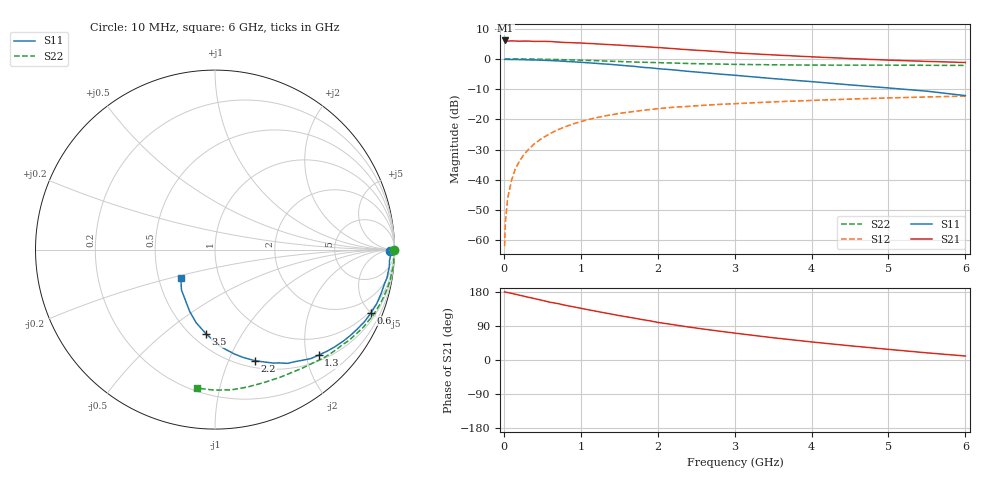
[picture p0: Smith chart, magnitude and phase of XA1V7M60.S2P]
! SIEMENS Discrete & RF Semiconductors
! BFY180
! Si NPN RF Bipolar Junction Transistor in MICRO-X
! VCE = 1.75 V  IC = 0.6 mA
! Common Emitter S-Parameters:  May  1997
# GHz  S  MA  R  50
!  f  S11  S21  S12  S22
! GHz  MAG  ANG  MAG  ANG  MAG  ANG  MAG  ANG
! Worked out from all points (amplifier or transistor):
!   36 points, 10 MHz to 6 GHz, reference 50 ohm
!   highest |S21| = 6.1 dB at 20 MHz (marker M1)
!   |S21| within 3 dB of that: start of sweep to 2.36 GHz
!   unconditionally stable (mu >= 1): 4.518 GHz to end of sweep
!   at 250 MHz: K = 0.07, MSG = 19.0 dB, |S12| = -32.0 dB
!   at 1.4 GHz: K = 0.44, MSG = 11.6 dB, |S12| = -18.5 dB
!   at 6 GHz: K = 1.05, MAG = 4.2 dB, |S12| = -12.3 dB
!   S11 on the Smith chart (normalised r, x): 10 MHz: 78, -23; 600 MHz: 0.86, -5.00; 1.3 GHz: 0.61, -2.24; 2.2 GHz: 0.57, -1.25; 3.5 GHz: 0.59, -0.71; 6 GHz: 0.65, -0.22
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0.01  0.9766 -0.4  1.98 179.8  0.0008 96.3  0.999 -0.2
0.02  0.9797 -0.6  2.015 179.1  0.002 94.2  0.9999 -0.6
0.05  0.979 -1.7  1.963 178.0  0.005 89.9  0.9982 -1.2
0.1  0.9742 -3.7  1.986 175.8  0.0098 86.7  0.9958 -2.4
0.15  0.976 -5.7  1.972 173.6  0.0152 85.8  0.9986 -3.7
0.3  0.964 -11.1  1.971 166.4  0.0299 81.2  0.9925 -7.2
0.4  0.9578 -14.6  1.946 162.0  0.0398 79.1  0.991 -9.6
0.6  0.9379 -22.0  1.937 152.5  0.058 73.6  0.9792 -14.3
0.9  0.8936 -32.3  1.847 140.6  0.084 65.3  0.9588 -21.0
1.1  0.8598 -39.0  1.798 132.5  0.0991 60.6  0.9411 -25.2
1.3  0.8241 -45.5  1.742 124.9  0.1132 55.8  0.9233 -29.4
1.5  0.7878 -51.4  1.688 117.2  0.1254 51.6  0.9052 -33.3
1.8  0.7252 -60.5  1.601 106.6  0.1406 46.3  0.8797 -38.5
2  0.6889 -65.6  1.541 99.3  0.1501 42.8  0.8664 -41.9
2.2  0.658 -70.2  1.478 93.3  0.1583 39.4  0.8532 -45.3
2.4  0.6207 -75.4  1.414 87.1  0.1639 36.6  0.8381 -48.2
2.8  0.561 -83.6  1.313 76.2  0.1769 31.6  0.8197 -53.8
3.5  0.4717 -96.1  1.163 58.7  0.1945 24.1  0.7981 -63.2
4  0.4204 -104.5  1.081 47.7  0.2054 19.3  0.7892 -69.8
4.5  0.3713 -112.4  1.013 37.5  0.2162 14.9  0.7869 -76.5
5.5  0.2921 -129.8  0.908 18.9  0.2344 6.2  0.7828 -90.4
6  0.2468 -140.5  0.871 10.5  0.2423 1.6  0.7781 -97.4
